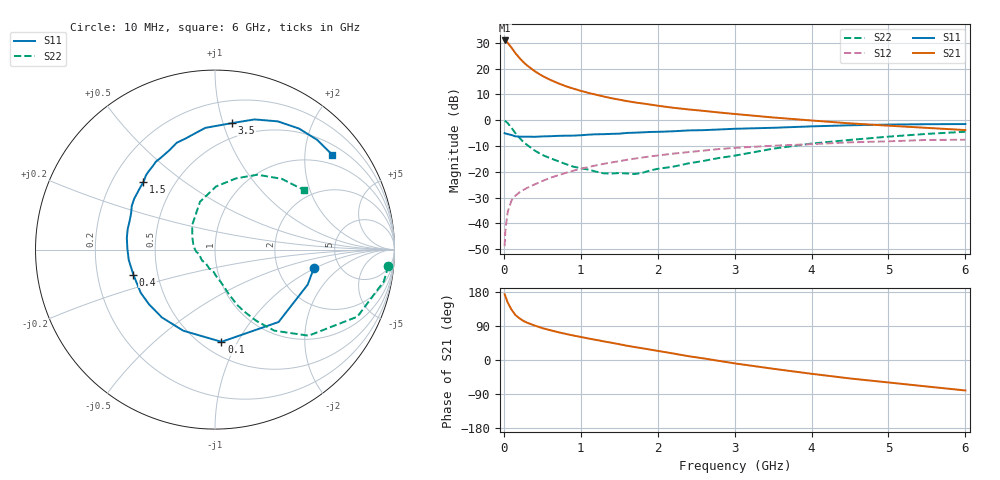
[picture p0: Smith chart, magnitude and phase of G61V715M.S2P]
! SIEMENS Small Signal Semiconductors
! BFG193
! Si NPN RF Bipolar Junction Transistor in SOT223
! VCE = 1.75 V  IC = 15 mA
! Common Emitter S-Parameters:  August  1996
# GHz  S  MA  R  50
!  f  S11  S21  S12  S22
! GHz  MAG  ANG  MAG  ANG  MAG  ANG  MAG  ANG
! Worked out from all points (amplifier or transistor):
!   36 points, 10 MHz to 6 GHz, reference 50 ohm
!   highest |S21| = 30.9 dB at 10 MHz (marker M1)
!   |S21| within 3 dB of that: start of sweep to 104.6 MHz
!   unconditionally stable (mu >= 1): 745.2 MHz to 2.729 GHz
!   at 250 MHz: K = 0.67, MSG = 24.9 dB, |S12| = -27.1 dB
!   at 1.4 GHz: K = 1.07, MAG = 10.9 dB, |S12| = -16.4 dB
!   at 6 GHz: K = 0.92, MSG = 1.9 dB, |S12| = -7.6 dB
!   S11 on the Smith chart (normalised r, x): 10 MHz: 3.24, -0.96; 100 MHz: 0.62, -0.86; 400 MHz: 0.36, -0.13; 1.5 GHz: 0.33, +0.36; 3.5 GHz: 0.38, +1.07; 6 GHz: 0.73, +2.64
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0.01  0.5607 -10.4  35.14 173.7  0.0036 87.2  0.9702 -5.4
0.02  0.5521 -20.7  34.62 168.5  0.0071 81.8  0.9572 -10.7
0.05  0.5369 -48.7  31.69 151.6  0.0166 71.5  0.8772 -25.2
0.1  0.5151 -86.0  25.43 132.9  0.0278 61.2  0.7085 -42.6
0.15  0.4853 -111.4  19.94 118.8  0.0342 54.7  0.5597 -53.8
0.2  0.48 -128.0  16.27 110.4  0.0395 53.5  0.4602 -59.8
0.25  0.4776 -140.4  13.54 103.6  0.044 52.4  0.3827 -64.7
0.3  0.4787 -149.9  11.59 98.6  0.0484 53.2  0.3331 -68.1
0.4  0.4759 -163.0  8.936 91.0  0.0567 54.1  0.2581 -72.9
0.5  0.484 -173.2  7.218 84.2  0.066 54.4  0.2118 -76.4
0.6  0.4883 179.3  6.084 78.8  0.0757 55.0  0.1838 -79.9
0.7  0.4956 172.4  5.245 73.7  0.0848 54.8  0.1615 -84.4
0.9  0.5017 161.5  4.105 64.7  0.1045 52.7  0.1258 -93.0
1.1  0.5236 152.4  3.377 56.8  0.1233 50.8  0.1101 -106.8
1.5  0.5474 136.8  2.505 41.7  0.1602 43.9  0.0943 -139.8
1.7  0.572 130.2  2.212 34.2  0.1796 40.4  0.0902 -158.6
2.2  0.6085 114.8  1.741 17.2  0.2242 29.7  0.1252 165.5
2.8  0.6597 99.1  1.407 -2.4  0.275 16.4  0.1852 133.6
3.5  0.7113 82.3  1.127 -23.1  0.3193 -0.5  0.2798 107.3
4.5  0.7956 63.9  0.867 -48.7  0.3715 -20.1  0.414 73.5
5.5  0.8352 47.1  0.709 -69.9  0.4133 -43.1  0.542 46.7
6  0.8403 39.0  0.642 -80.4  0.417 -56.2  0.5956 33.9
